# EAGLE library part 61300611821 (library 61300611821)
WURTH ELEKTRONIK - 61300611821 - PCB Receptacle, Board-to-Board, 2.54 mm, 1 Rows, 6 Contacts, Through Hole, WR-PHD Series Source: Datasheet
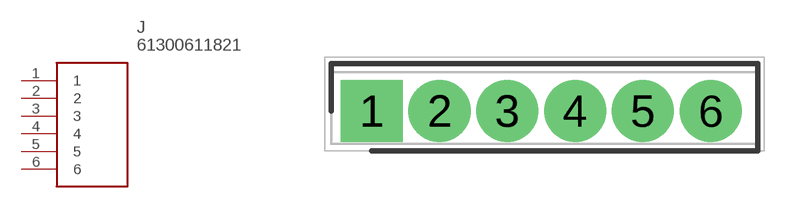
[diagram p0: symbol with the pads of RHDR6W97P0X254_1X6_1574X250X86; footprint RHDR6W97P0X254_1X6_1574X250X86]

Designator prefix J

## 61300611821 (Description: WURTH ELEKTRONIK - 61300611821 - PCB Receptacle, Board-to-Board, 2.54 mm, 1 Rows, 6 Contacts, Through Hole, WR-PHD Series; Height: 8.65mm; Manufacturer_Name: Wurth Elektronik; Manufacturer_Part_Number: 61300611821; Mouser_Part_Number: 710-61300611821; Mouser_Price-Stock: https://www.mouser.co.uk/ProductDetail/Wurth-Elektronik/61300611821?qs=iLbezkQI%252BsgS21jF2eozhA%3D%3D)  [RHDR6W97P0X254_1X6_1574X250X86]
1  1
2  2
3  3
4  4
5  5
6  6

## Footprint RHDR6W97P0X254_1X6_1574X250X86 (pad centres in mm)
DDTC113ZCA
drill 1.55 pad 2.325 square: 1 0,0
drill 1.55 pad 2.325: 2 2.54,0; 3 5.08,0; 4 7.62,0; 5 10.16,0; 6 12.7,0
